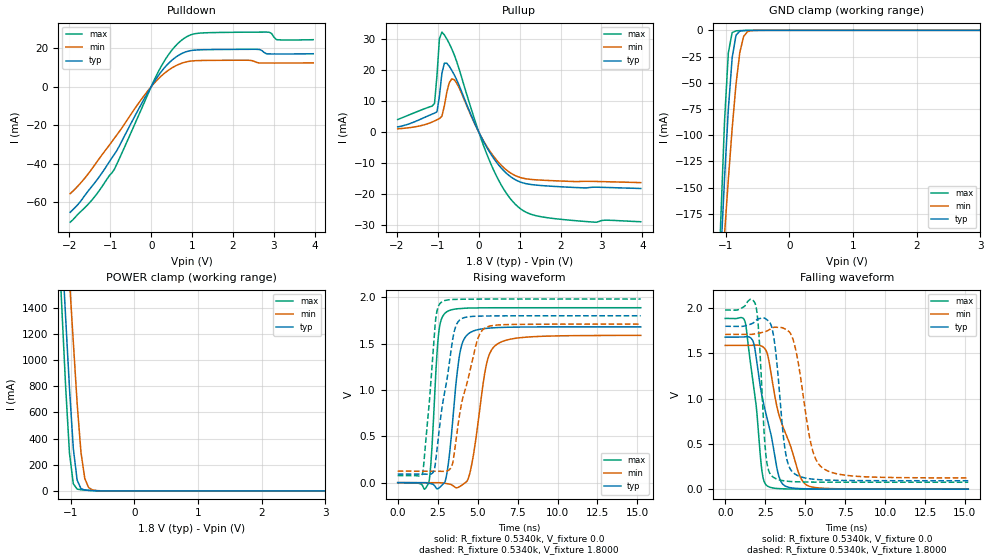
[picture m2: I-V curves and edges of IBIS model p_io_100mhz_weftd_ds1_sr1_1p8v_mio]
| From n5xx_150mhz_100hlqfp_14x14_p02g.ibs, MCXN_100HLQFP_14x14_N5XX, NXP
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[Model] p_io_100mhz_weftd_ds1_sr1_1p8v_mio
|   Model p_io_100mhz_weftd_ds1_sr1_1p8v_mio
| This model was characterised for following simulation conditions:
| External (pad) voltage:
|   - Typ: 1.8V,   - Min: 1.71V,   - Max: 1.98V
| Library cells for typ/min/max conditions are connected as defined below:
|  pad - External Pad
|  ipp_do_lv - Core Input
|  ipp_obe_lv - Output Buffer Enable
|  IOGC - NC
|  REFH3V3 - REFH3V3
|  REFL3V3 - REFL3V3
|  ZI - NC
|  abut_ncal_vddio[1] - vssio vddio vddio
|  abut_ncal_vddio[2] - vddio vddio vssio
|  abut_ncal_vddio[3] - vddio
|  abut_ncal_vddio[4] - vssio vddio vddio
|  abut_ncal_vddio[5] - vddio vddio vssio
|  abut_ncal_vddio[6] - vddio
|  abut_pcal_vddio[1] - vssio
|  abut_pcal_vddio[2] - vddio vssio vddio
|  abut_pcal_vddio[3] - vssio
|  abut_pcal_vddio[4] - vssio
|  abut_pcal_vddio[5] - vddio vssio vddio
|  abut_pcal_vddio[6] - vssio
|  ipp_do_1p8v - ipp_do_1p8v
|  ipp_dse_lv - vdd_lv
|  ipp_eftd_lv - NC
|  ipp_ina_mux_vddio - NC
|  ipp_ina_mux_vddio[0] - NC
|  ipp_ina_mux_vddio[1] - NC
|  ipp_ina_r0_vddio - NC
|  ipp_ina_r0a_vddio - NC
|  ipp_ina_r0b_vddio - NC
|  ipp_ina_r0c_vddio - NC
|  ipp_ina_r0d_vddio - NC
|  ipp_ina_r0e_vddio - NC
|  ipp_ina_r0f_vddio - NC
|  ipp_ina_r300_vddio - NC
|  ipp_ina_r300a_vddio - NC
|  ipp_ina_r300b_vddio - NC
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Model_type I/O
Polarity   Non-Inverting
Enable   Active-High
Vinl =   0.5400V
Vinh =   1.2600V
Vmeas =  0.9000V
Cref =   30.0000pF
Rref =   1.0000M
Vref =   1.8000V
C_comp   1.4209pF   1.3571pF   1.5007pF
|C_comp_pullup   0.7326pF   0.7591pF   0.7066pF
|C_comp_pulldown   0.6105pF   0.6615pF   0.5696pF
[Model Spec]
| variable   typ   min   max
Vinh   1.2600V   1.1970V   1.3860V
Vinl   0.5400V   0.5130V   0.5940V
[Temperature Range]   25.0000   0.1250k   -40.0000
[Voltage Range]   1.8000V   1.7100V   1.9800V
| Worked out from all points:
|   slope of the pulldown table from 0 to 0.27 V, typ, clamps not added: 32.1 ohm
|   slope of the pullup table from 0 to 0.27 V, typ, clamps not added: 40.9 ohm
|   GND clamp passes 1 mA (typ) near -0.78 V on its own axis
|   POWER clamp passes 1 mA (typ) near -0.56 V on its own axis
|   rising waveform, R_fixture 0.5340k, V_fixture 0.0: 20-80 % time 580ps typ, 790ps min, 363ps max; typ from 0 V to 1.68 V
|   rising waveform, R_fixture 0.5340k, V_fixture 1.8000: 20-80 % time 860ps typ, 1.14ns min, 527ps max; typ from 0.093 V to 1.8 V
|   falling waveform, R_fixture 0.5340k, V_fixture 0.0: 20-80 % time 1.11ns typ, 1.48ns min, 698ps max; typ from 1.68 V to 0 V
|   falling waveform, R_fixture 0.5340k, V_fixture 1.8000: 20-80 % time 551ps typ, 874ps min, 353ps max; typ from 1.8 V to 0.093 V
[Pulldown]
|Voltage   I(typ)   I(min)   I(max)
-1.98V    -65.1mA    -55.47mA   -70.23mA
-1.44V    -51.41mA   -42.35mA   -58.53mA
-900mV    -35.03mA   -26.74mA   -42.82mA
-240mV    -8.989mA   -6.551mA   -11.62mA
180mV     5.908mA    4.185mA    8mA
480mV     13.23mA    9.376mA    18.23mA
780mV     17.5mA     12.4mA     24.7mA
1.2V      19.1mA     13.55mA    27.77mA
2.58V     19.36mA    12.56mA    28.27mA
2.82V     17.02mA    12.25mA    28.29mA
3.06V     16.94mA    12.25mA    24.4mA
3.96V     17.07mA    12.34mA    24.35mA
[Pullup]
|Voltage   I(typ)   I(min)   I(max)
-1.98V    1.629mA    999.6uA    4.015mA
-1.08V    6.088mA    3.551mA    9.212mA
-1.02V    6.511mA    3.928mA    18.3mA
-960mV    11.61mA    4.321mA    30.17mA
-900mV    18.93mA    5.074mA    32.31mA
-840mV    22.23mA    8.425mA    31.4mA
-720mV    21.25mA    15.95mA    28.6mA
-600mV    18.53mA    16.91mA    25.01mA
240mV     -5.966mA   -5.551mA   -8.574mA
900mV     -15.51mA   -14.17mA   -23.49mA
1.68V     -17.49mA   -15.7mA    -27.77mA
3.96V     -18.31mA   -16.4mA    -29.07mA
[GND_clamp]
|Voltage   I(typ)   I(min)   I(max)
-1.98V    -1.543A    -1.201A    -2.023A
-1.14V    -295.8mA   -306.3mA   -290.9mA
-1.08V    -216.4mA   -249.6mA   -182.7mA
-1.02V    -141.5mA   -194.6mA   -86.96mA
-960mV    -75.17mA   -142.1mA   -21.27mA
-900mV    -26.1mA    -93.57mA   -2.203mA
-840mV    -4.74mA    -51.67mA   -459.1uA
-780mV    -724.6uA   -21.14mA   -268.2uA
-720mV    -210.5uA   -5.843mA   -184.1uA
-660mV    -110.6uA   -1.28mA    -119.5uA
-420mV    -5.355uA   -12.87uA   -3.609uA
3.96V     0A         0A         0A
[POWER_clamp]
|Voltage   I(typ)   I(min)   I(max)
-1.98V    9.578A     9.289A     10.07A
-1.2V     2.41A      3.038A     2.007A
-1.14V    1.864A     2.561A     1.396A
-1.08V    1.321A     2.084A     791.3mA
-1.02V    783mA      1.609A     287.7mA
-960mV    325.3mA    1.137A     54.76mA
-900mV    82.69mA    671.2mA    14.16mA
-840mV    18.08mA    297mA      8.834mA
-780mV    6.944mA    95.27mA    6.398mA
-720mV    4.174mA    26.01mA    4.41mA
-660mV    2.65mA     7.951mA    2.754mA
3.96V     0A         0A         0A
[Ramp]
| variable   typ   min   max
dV/dt_r  1.0081/0.5805n   0.9529/0.7899n   1.1320/0.3630n
dV/dt_f  1.0242/0.5508n   0.9513/0.8738n   1.1422/0.3535n
R_load = 0.5340k
[Rising Waveform]
R_fixture= 0.5340k
V_fixture= 0.0
V_fixture_min= 0.0
V_fixture_max= 0.0
|time   V(typ)   V(min)   V(max)
0s        469.4pV    172.1nV    14.64pV
1.946ns   -6.031mV   159.3uV    1.054mV
2.121ns   -12.62mV   403.3uV    315.1mV
2.543ns   -62.32mV   25.91uV    1.58V
3.062ns   82.87mV    -9.851mV   1.842V
3.847ns   1.353V     -45.77mV   1.877V
4.433ns   1.607V     53.33mV    1.883V
5.526ns   1.664V     1.254V     1.886V
6.1ns     1.671V     1.477V     1.886V
15.21ns   1.68V      1.588V     1.887V
[Rising Waveform]
R_fixture= 0.5340k
V_fixture= 1.8000
V_fixture_min= 1.7100
V_fixture_max= 1.9800
|time   V(typ)   V(min)   V(max)
0s        93mV       124mV      76.32mV
1.558ns   93.31mV    123.9mV    104.9mV
1.967ns   89.07mV    124.2mV    837.6mV
2.353ns   200.5mV    124.1mV    1.728V
2.748ns   779.3mV    121.6mV    1.949V
3.386ns   1.485V     179.8mV    1.975V
3.681ns   1.706V     503.7mV    1.977V
4.887ns   1.795V     1.478V     1.98V
5.41ns    1.797V     1.662V     1.98V
15.21ns   1.8V       1.71V      1.98V
[Falling Waveform]
R_fixture= 0.5340k
V_fixture= 0.0
V_fixture_min= 0.0
V_fixture_max= 0.0
|time   V(typ)   V(min)   V(max)
0s        1.68V      1.588V     1.887V
1.257ns   1.684V     1.588V     1.84V
1.786ns   1.612V     1.592V     1.127V
1.957ns   1.431V     1.593V     891.7mV
2.307ns   1.024V     1.578V     189.4mV
2.618ns   783.7mV    1.505V     37.56mV
3.502ns   78.97mV    743.4mV    4.489mV
4.623ns   6.822mV    166.3mV    876.3uV
5.045ns   3.898mV    50.88mV    548.2uV
15.21ns   36.63uV    86.83uV    22.7uV
[Falling Waveform]
R_fixture= 0.5340k
V_fixture= 1.8000
V_fixture_min= 1.7100
V_fixture_max= 1.9800
|time   V(typ)   V(min)   V(max)
0s        1.8V       1.71V      1.98V
1.901ns   1.859V     1.716V     2.038V
2.115ns   1.885V     1.724V     1.694V
2.548ns   1.881V     1.743V     373mV
3.02ns    1.7V       1.788V     130.7mV
3.76ns    420mV      1.769V     90.15mV
4.345ns   169mV      1.591V     82.22mV
5.38ns    112.9mV    489.1mV    78.03mV
6.075ns   102.8mV    236.4mV    77.16mV
15.21ns   93.06mV    124.4mV    76.35mV
